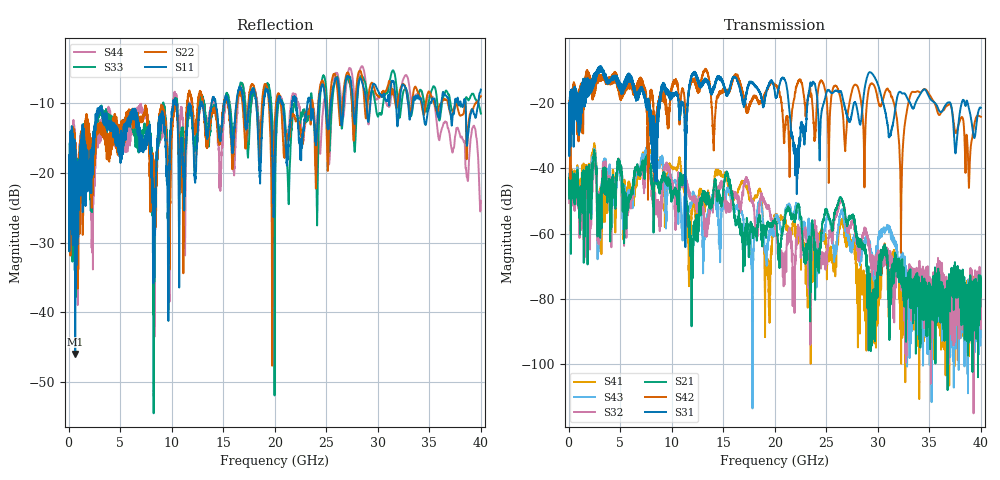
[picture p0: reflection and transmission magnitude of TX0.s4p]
!Agilent Technologies,N5245A,MY49151084,A.09.00.04
!Agilent N5245A: A.09.00.04
!Date: Thursday, January 20, 2011 08:51:13
!Correction: S11(Full 4 Port(1,2,3,4))
!S12(Full 4 Port(1,2,3,4))
!S13(Full 4 Port(1,2,3,4))
!S14(Full 4 Port(1,2,3,4))
!S21(Full 4 Port(1,2,3,4))
!S22(Full 4 Port(1,2,3,4))
!S23(Full 4 Port(1,2,3,4))
!S24(Full 4 Port(1,2,3,4))
!S31(Full 4 Port(1,2,3,4))
!S32(Full 4 Port(1,2,3,4))
!S33(Full 4 Port(1,2,3,4))
!S34(Full 4 Port(1,2,3,4))
!S41(Full 4 Port(1,2,3,4))
!S42(Full 4 Port(1,2,3,4))
!S43(Full 4 Port(1,2,3,4))
!S44(Full 4 Port(1,2,3,4))
!S4P File: Measurements: <S11,S12,S13,S14>,
!<S21,S22,S23,S24>,
!<S31,S32,S33,S34>,
!<S41,S42,S43,S44>:
# Hz S  dB  R 50
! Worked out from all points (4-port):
!   3996 points, 50 MHz to 40 GHz, reference 50 ohm
!   strongest paths, dB at 50 MHz, 10.04 GHz, 20.03 GHz, 30.02 GHz, 40 GHz:
!     S31: -22.1, -17.3, -17.2, -14.3, -21.4
!     S42: -22.7, -14.9, -14.4, -19.2, -24.2
!     S21: -49.2, -47.9, -55.7, -73.1, -76.4
!     S32: -50.6, -45.1, -56.9, -66.5, -89.1
!     S43: -47.5, -44.0, -55.9, -62.3, -81.6
!     S41: -48.2, -40.0, -55.0, -87.5, -78.4
!   lowest |S11| = -46.0 dB at 640 MHz (marker M1), VSWR 1.01, Z = 49.5 + j0.159 ohm
!   |S11| at or under -10 dB: start of sweep to 10.14 GHz; 10.42 GHz to 11.7 GHz (1.278 GHz wide, 11.6 % of centre); 38.52 GHz to 39.74 GHz (1.227 GHz wide, 3.14 % of centre)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
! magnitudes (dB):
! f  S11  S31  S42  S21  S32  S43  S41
! 50 MHz  -18.6  -22.1  -22.7  -49.2  -50.6  -47.5  -48.2
! 640 MHz  -46.0  -22.0  -23.1  -45.2  -46.3  -44.8  -43.5
! 23.39 GHz  -9.5  -15.2  -15.8  -69.6  -69.7  -58.7  -64.6
! 26.41 GHz  -11.9  -16.4  -19.2  -48.9  -50.5  -53.9  -56.7
! 29.45 GHz  -7.7  -10.9  -13.9  -86.4  -68.0  -66.1  -82.0
! 32.26 GHz  -8.0  -16.7  -54.0  -70.2  -69.5  -70.6  -99.9
! 40 GHz  -8.0  -21.4  -24.2  -76.4  -89.1  -81.6  -78.4
